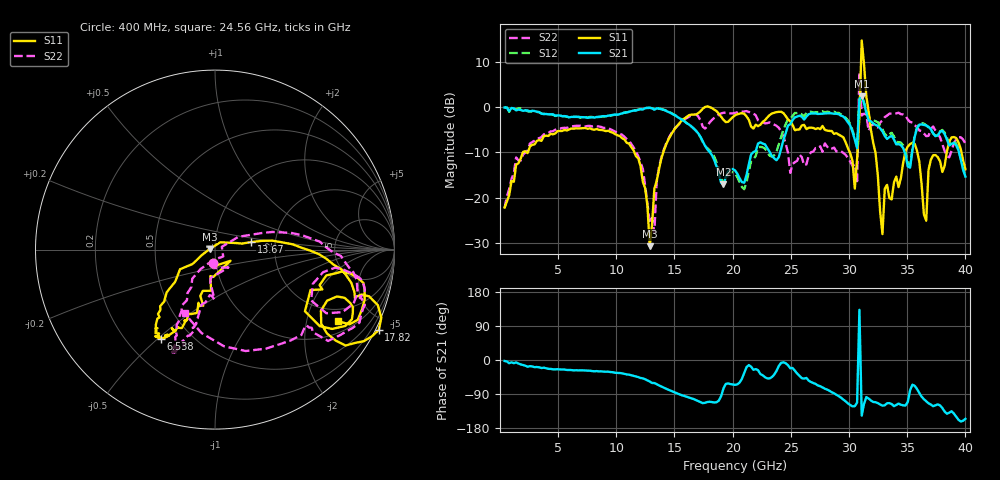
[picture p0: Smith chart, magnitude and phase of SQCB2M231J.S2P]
! Network Analyzer HP8722ES.07.66: Jul 25, 2000 Serial No. US39175408
! 27 Oct 2004  13:35:27
! Frequency  S11  S21  S12  S22
# HZ  S  DB R  50
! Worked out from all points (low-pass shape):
!   201 points, 400 MHz to 40 GHz, reference 50 ohm
!   highest |S21| = 2.39 dB at 31.09 GHz (marker M1); lowest = -17.1 dB at 19.21 GHz (marker M2)
!   |S21| within 3 dB of the highest: 11.89 GHz to 14.04 GHz (2.156 GHz wide, 16.6 % of centre); 30.85 GHz to 31.43 GHz (578.6 MHz wide, 1.86 % of centre)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
!   lowest |S11| = -30.7 dB at 12.87 GHz (marker M3), VSWR 1.06, Z = 47.2 + j0.362 ohm
!   |S11| at or under -10 dB: 11.55 GHz to 14.04 GHz (2.482 GHz wide, 19.4 % of centre); 32.26 GHz to 34.83 GHz (2.563 GHz wide, 7.64 % of centre); 35.87 GHz to 38.4 GHz (2.531 GHz wide, 6.82 % of centre)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
!   |S22| runs from -27.7 to 7.6 dB; largest |S21 - S12| = 0.3
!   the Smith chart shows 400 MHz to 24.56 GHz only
!   S11 on the Smith chart (normalised r, x): 400 MHz: 0.96, -0.15; 6.538 GHz: 0.34, -0.51; 13.67 GHz: 1.49, +0.13; 17.82 GHz: -0.16, -4.30; 24.56 GHz: 1.43, -3.11
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4e8  -22.18 -100.1  -0.11 -2.7  -0.07 -2.2  -22.32 -96.4
6.538e9  -4.70 -121.2  -2.18 -27.1  -2.15 -26.6  -4.15 -111.8
7.132e9  -4.66 -123.5  -2.26 -27.3  -2.37 -28.1  -4.25 -111.2
1.1884e10  -11.34 -142.8  -0.61 -45.1  -0.56 -44.9  -10.85 -122.3
1.2874e10  -30.73 172.4  -0.19 -56.8  -0.16 -57.2  -25.64 -83.5
1.3666e10  -13.79 11.7  -0.37 -67.1  -0.34 -67.4  -13.37 22.5
1.7824e10  0.14 -26.1  -9.35 -110.9  -9.08 -108.9  -4.22 -11.8
1.921e10  -2.83 -34.9  -17.09 -74.9  -16.93 -88.1  -1.27 -15.0
2.02e10  -1.83 -21.5  -14.00 -65.6  -14.71 -68.9  -1.29 -18.5
2.4556e10  -1.99 -30.1  -5.78 -8.4  -3.81 -10.1  -8.09 -115.5
2.6932e10  -4.62 -14.4  -1.43 -60.9  -1.25 -62.6  -9.80 65.2
3.0694e10  -11.43 46.9  -9.09 -112.5  -8.70 -112.1  -16.37 -106.5
3.0892e10  -2.08 0.7  1.72 132.4  1.89 146.4  7.61 14.6
3.109e10  14.70 -79.6  2.39 -146.8  2.45 -146.3  -1.87 163.4
3.1288e10  9.55 -97.8  0.81 -115.9  1.06 -114.7  -1.49 -145.4
3.1486e10  2.35 -91.3  -1.20 -97.9  -0.71 -96.5  -1.65 -126.9
3.1684e10  -0.99 -119.4  -2.96 -101.8  -2.34 -102.9  -5.26 -140.3
3.2872e10  -28.06 -34.0  -5.40 -120.5  -4.93 -123.4  -2.93 179.7
3.3466e10  -20.11 -135.1  -6.61 -113.7  -6.00 -117.1  -1.48 165.4
3.6634e10  -25.10 144.2  -4.07 -109.0  -4.05 -112.8  -6.42 133.1
3.8218e10  -12.98 44.7  -5.98 -136.1  -5.64 -136.6  -9.70 32.5
4e10  -13.74 -85.1  -15.35 -155.2  -15.50 -158.9  -8.06 -149.8
